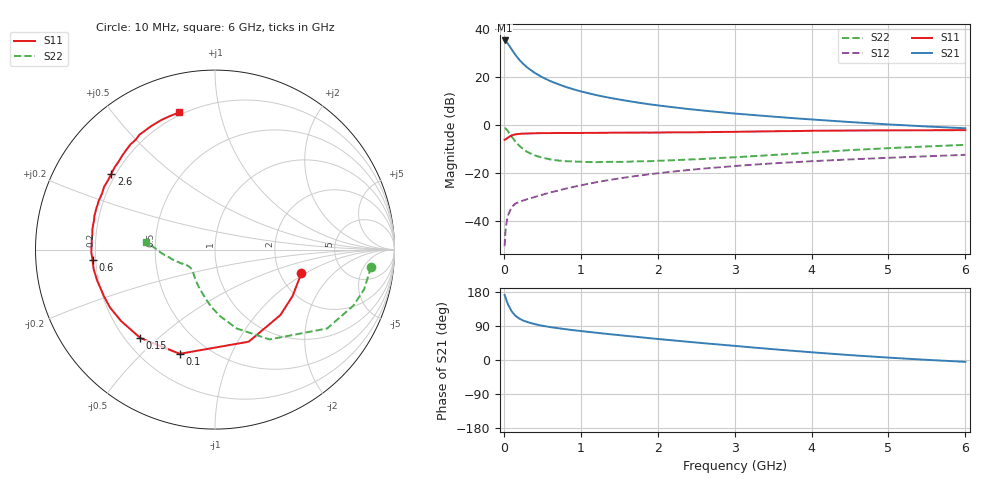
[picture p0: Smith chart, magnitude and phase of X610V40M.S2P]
! SIEMENS Small Signal Semiconductors
! BFP193W
! Si NPN RF Bipolar Junction Transistor in SOT343
! VCE = 10 V  IC = 40 mA
! Common Emitter S-Parameters:  April 1994
# GHz  S  MA  R  50
!  f  S11  S21  S12  S22
! GHz  MAG  ANG  MAG  ANG  MAG  ANG  MAG  ANG
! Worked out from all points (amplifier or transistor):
!   40 points, 10 MHz to 6 GHz, reference 50 ohm
!   highest |S21| = 35.4 dB at 10 MHz (marker M1)
!   |S21| within 3 dB of that: start of sweep to 86.66 MHz
!   unconditionally stable (mu >= 1): 795.3 MHz to 5.049 GHz
!   at 200 MHz: K = 0.48, MSG = 29.7 dB, |S12| = -32.0 dB
!   at 1.5 GHz: K = 1.10, MAG = 14.5 dB, |S12| = -22.2 dB
!   at 6 GHz: K = 0.96, MSG = 5.5 dB, |S12| = -12.4 dB
!   S11 on the Smith chart (normalised r, x): 10 MHz: 2.63, -0.92; 100 MHz: 0.35, -0.66; 150 MHz: 0.26, -0.44; 600 MHz: 0.19, -0.04; 2.6 GHz: 0.18, +0.32; 6 GHz: 0.19, +0.75
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0.01  0.4991 -15.2  58.57 171.6  0.003 70.7  0.8749 -6.3
0.02  0.5037 -30.9  57.61 166.1  0.0058 68.9  0.8599 -14.9
0.03  0.5155 -45.0  55.82 159.9  0.0082 69.7  0.8321 -22.0
0.05  0.5464 -69.9  50.94 148.6  0.0127 61.5  0.7639 -35.1
0.1  0.6129 -108.7  38.47 128.9  0.0194 49.5  0.5857 -58.7
0.15  0.6447 -130.2  29.37 116.8  0.0232 43.6  0.4557 -74.6
0.2  0.6576 -142.8  23.23 109.4  0.0251 42.9  0.373 -85.5
0.25  0.6682 -151.2  19.19 104.2  0.0269 42.3  0.3199 -93.7
0.3  0.6708 -157.0  16.19 100.5  0.0285 43.5  0.2793 -100.6
0.4  0.6789 -165.3  12.39 94.7  0.0318 45.6  0.2353 -111.0
0.5  0.6849 -170.9  10.01 90.4  0.0354 48.7  0.2105 -118.9
0.6  0.6848 -175.2  8.37 86.9  0.0395 50.8  0.1941 -125.1
0.8  0.6879 178.2  6.329 81.3  0.0474 54.6  0.1778 -133.1
1.1  0.6922 170.8  4.646 74.2  0.0601 56.9  0.1706 -141.2
1.3  0.6935 166.4  3.937 69.7  0.0689 57.6  0.1711 -144.0
1.6  0.7 160.8  3.229 63.5  0.082 57.6  0.1725 -147.3
2.2  0.7101 150.3  2.371 51.8  0.1078 55.3  0.1858 -153.4
2.6  0.7156 143.8  2.015 44.3  0.1247 53.0  0.1981 -157.0
3.2  0.7364 134.4  1.653 33.7  0.1486 49.0  0.2244 -162.7
4.5  0.7743 117.5  1.165 12.9  0.1936 39.7  0.3024 -176.7
5.5  0.7848 109.0  0.941 0.4  0.2249 33.4  0.3606 176.0
6  0.7899 104.7  0.863 -4.9  0.2411 30.8  0.3893 173.4
